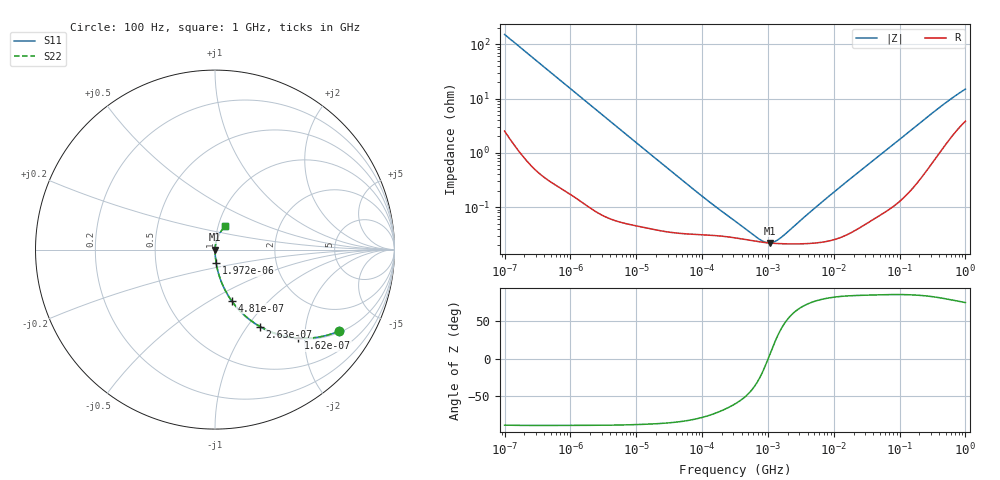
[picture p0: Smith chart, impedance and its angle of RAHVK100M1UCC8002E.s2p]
! RAHVK100M1UCC8002E  S-PARAMETER MODEL  (AEC-Q200 qualified)
! Model Generated by ELNA Corporation (http://www.ty-top.com)
! Version 1.0
! ELNA Control No. 201214
! Copyright (c) 2020 ELNA CO.,LTD. All Rights Reserved.
! Products Name : CONDUCTIVE POLYMER HYBRID ALUMINUM ELECTROLYTIC CAPACITORS
! Characteristics :
!  Capacitance  :  10uF  ,  Rated voltage  :  50V
!  Operating Temp. Range  :  -55 to +125 degC  ,  Endurance  :  4000hr at 125 degC
!  Dimension D  :  5mm  ,  Dimension L  :  5.8mm
! Frequency Range : 100Hz - 1GHz
! External Node Assignments :
!  1  o---| |---o  2
# MHz S RI R 50
!Freq[MHz].  S11 Real  S11 Imag  S21 Real  S21 Imag  S12 Real  S12 Imag  S22 Real  S22 Imag
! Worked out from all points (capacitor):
!   401 points, 100 Hz to 1 GHz, reference 50 ohm
!   read as one part in series: C = 10.5 uF near 108 Hz
!   lowest |Z| = 22 mohm at 1.059 MHz (marker M1)
!   series resonance near 1.01 MHz, so ESL is about 2.4 nH
!   S11 on the Smith chart (normalised r, x): 100 Hz: 1.05, -3.02; 162 Hz: 1.02, -1.86; 263 Hz: 1.01, -1.15; 481 Hz: 1.01, -0.63; 1.972 kHz: 1.00, -0.15; 1 GHz: 1.08, +0.29
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0.0001  0.6924 -0.4533  0.3076 0.4533  0.3076 0.4533  0.6924 -0.4533
0.000162  0.4651 -0.4929  0.5349 0.4929  0.5349 0.4929  0.4651 -0.4929
0.000263  0.2504 -0.4285  0.7496 0.4285  0.7496 0.4285  0.2504 -0.4285
0.000363  0.1502 -0.3527  0.8498 0.3527  0.8498 0.3527  0.1502 -0.3527
0.000481  0.0922 -0.2846  0.9078 0.2846  0.9078 0.2846  0.0922 -0.2846
0.000846  0.033 -0.1732  0.967 0.1732  0.967 0.1732  0.033 -0.1732
0.001488  0.0116 -0.1011  0.9884 0.1011  0.9884 0.1011  0.0116 -0.1011
0.001972  0.00691 -0.0768  0.9931 0.0768  0.9931 0.0768  0.00691 -0.0768
0.005188  0.00142 -0.0295  0.9986 0.0295  0.9986 0.0295  0.00142 -0.0295
0.022131  0.000421 -0.00699  0.9996 0.00699  0.9996 0.00699  0.000421 -0.00699
0.106537  0.000311 -0.00147  0.9997 0.00147  0.9997 0.00147  0.000311 -0.00147
0.316228  0.000272 -0.000484  0.9997 0.000484  0.9997 0.000484  0.000272 -0.000484
0.737055  0.00023 -0.000117  0.9998 0.000117  0.9998 0.000117  0.00023 -0.000117
0.901571  0.000223 -4.2e-05  0.9998 4.2e-05  0.9998 4.2e-05  0.000223 -4.2e-05
1.059254  0.000219 1.79e-05  0.9998 -1.79e-05  0.9998 -1.79e-05  0.000219 1.79e-05
1.295687  0.000215 9.48e-05  0.9998 -9.48e-05  0.9998 -9.48e-05  0.000215 9.48e-05
1.584893  0.000212 0.000176  0.9998 -0.000176  0.9998 -0.000176  0.000212 0.000176
4.704354  0.000217 0.000849  0.9998 -0.000849  0.9998 -0.000849  0.000217 0.000849
69.9842  0.00107 0.0124  0.9989 -0.0124  0.9989 -0.0124  0.00107 0.0124
412.0975  0.0148 0.0673  0.9852 -0.0673  0.9852 -0.0673  0.0148 0.0673
695.825  0.034 0.1026  0.966 -0.1026  0.966 -0.1026  0.034 0.1026
1000  0.0551 0.1313  0.9449 -0.1313  0.9449 -0.1313  0.0551 0.1313
